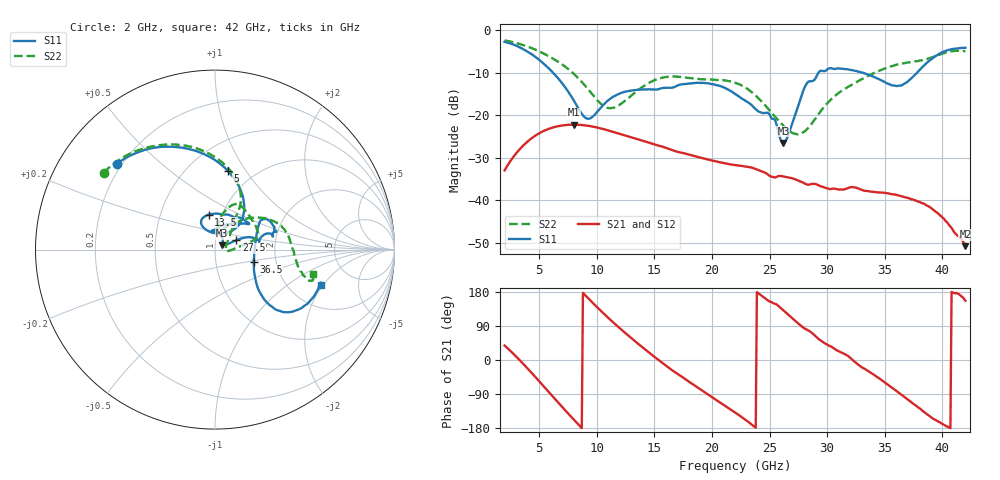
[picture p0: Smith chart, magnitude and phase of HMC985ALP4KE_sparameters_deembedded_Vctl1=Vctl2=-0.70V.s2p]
!s2p File: Measurements: S11, S21, S12, S22
# GHz S dB R 50.0
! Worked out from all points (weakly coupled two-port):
!   401 points, 2 GHz to 42 GHz, reference 50 ohm
!   highest |S21| = -22.25 dB at 8 GHz (marker M1); lowest = -50.8 dB at 42 GHz (marker M2)
!   lowest |S11| = -26.6 dB at 26.2 GHz (marker M3), VSWR 1.10, Z = 54.1 + j2.63 ohm
!   |S11| at or under -10 dB: 6.193 GHz to 29.26 GHz (23.07 GHz wide, 130 % of centre); 33.04 GHz to 37.81 GHz (4.772 GHz wide, 13.5 % of centre)
!   |S22| runs from -24.6 to -2.4 dB; largest |S21 - S12| = 0.00012
!   S11 on the Smith chart (normalised r, x): 2 GHz: 0.18, +0.36; 5 GHz: 0.76, +0.83; 13.5 GHz: 0.87, +0.35; 27.5 GHz: 1.26, +0.13; 36.5 GHz: 1.53, -0.21; 42 GHz: 2.97, -1.88
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2  -2.76 138.9  -33.03 38.1  -33.02 38.1  -2.45 145.4
3.4  -4.19 112.0  -27.78 -3.2  -27.78 -3.2  -3.35 122.8
5  -7.01 81.0  -24.29 -56.0  -24.29 -56.0  -5.01 98.2
6.4  -10.61 56.5  -22.77 -103.8  -22.78 -103.8  -7.04 78.5
8  -16.55 47.2  -22.25 -157.1  -22.26 -157.1  -10.29 62.0
8.7  -19.72 60.8  -22.34 -179.6  -22.35 -179.6  -12.22 58.4
9.5  -20.68 93.4  -22.64 155.4  -22.64 155.4  -14.77 58.4
11  -16.50 118.3  -23.62 111.1  -23.62 111.1  -18.34 73.8
13.5  -14.06 100.2  -25.64 45.1  -25.65 45.0  -14.31 79.1
15.4  -13.86 74.3  -27.21 -0.6  -27.22 -0.6  -11.42 68.3
18.9  -12.45 37.9  -29.96 -75.6  -29.95 -75.6  -11.53 40.7
22  -14.97 54.2  -31.76 -138.3  -31.76 -138.3  -12.38 15.8
24.9  -19.52 94.5  -34.07 156.2  -34.07 156.2  -18.59 4.1
26.2  -26.56 31.1  -34.45 130.6  -34.46 130.7  -22.52 -5.6
27.5  -17.75 23.5  -35.43 96.0  -35.45 96.0  -24.48 3.2
28.7  -12.01 10.5  -36.19 70.9  -36.20 71.0  -21.87 31.3
31  -9.03 21.2  -37.50 23.4  -37.51 23.2  -14.79 51.2
33.3  -10.24 32.5  -37.83 -24.1  -37.82 -24.3  -11.17 39.9
35.4  -12.75 11.2  -38.51 -67.8  -38.52 -68.0  -8.68 24.7
36.5  -12.97 -17.2  -39.14 -92.7  -39.15 -92.9  -7.87 15.9
39.6  -5.82 -42.7  -43.10 -161.5  -43.12 -162.1  -5.93 -15.5
42  -4.16 -18.4  -50.85 156.3  -50.83 157.9  -4.96 -14.1
